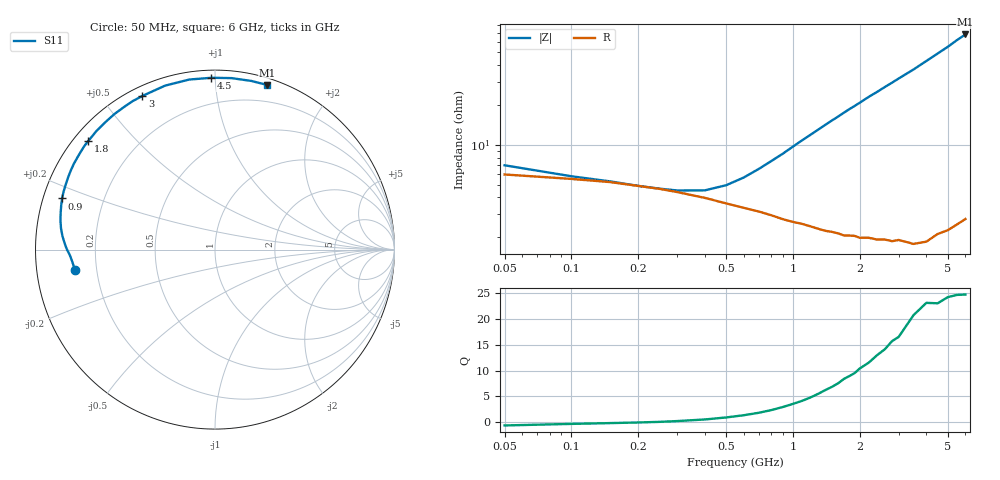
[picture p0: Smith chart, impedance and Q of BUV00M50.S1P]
! Infineon Technologies  Discrete & RF Semiconductors
! BB 833
! Si Tuning Diode in SOD323
! VR =
! S-Parameters:  June  1999
# GHz  S  MA  R  50
!  f  S11
! GHz  MAG  ANG
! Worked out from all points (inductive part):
!   34 points, 50 MHz to 6 GHz, reference 50 ohm
!   read as one part to ground: L = 1.56 nH near 1 GHz
!   highest Q = 24.8 at 6 GHz (marker M1), where L = 1.81 nH
!   S11 on the Smith chart (normalised r, x): 50 MHz: 0.12, -0.07; 900 MHz: 0.05, +0.16; 1.8 GHz: 0.04, +0.37; 3 GHz: 0.04, +0.63; 4.5 GHz: 0.04, +0.98; 6 GHz: 0.06, +1.36
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0.05  0.7877 -171.5
0.1  0.8012 -176.0
0.15  0.8108 -178.1
0.2  0.8217 -179.6
0.3  0.8384 177.6
0.4  0.853 175.0
0.5  0.8659 172.2
0.6  0.8757 169.5
0.8  0.8911 164.1
0.9  0.8985 161.5
1.1  0.9077 156.2
1.3  0.9165 151.2
1.4  0.9202 148.7
1.6  0.9254 144.0
1.7  0.9289 141.6
1.8  0.93 139.3
2  0.9344 135.0
2.2  0.9365 130.6
2.4  0.9404 126.7
2.6  0.9424 122.7
2.8  0.946 119.0
3  0.9469 115.3
3.5  0.955 106.9
4  0.9582 98.6
4.5  0.9576 91.2
5  0.9598 84.5
5.5  0.9612 77.9
6  0.9622 72.5
